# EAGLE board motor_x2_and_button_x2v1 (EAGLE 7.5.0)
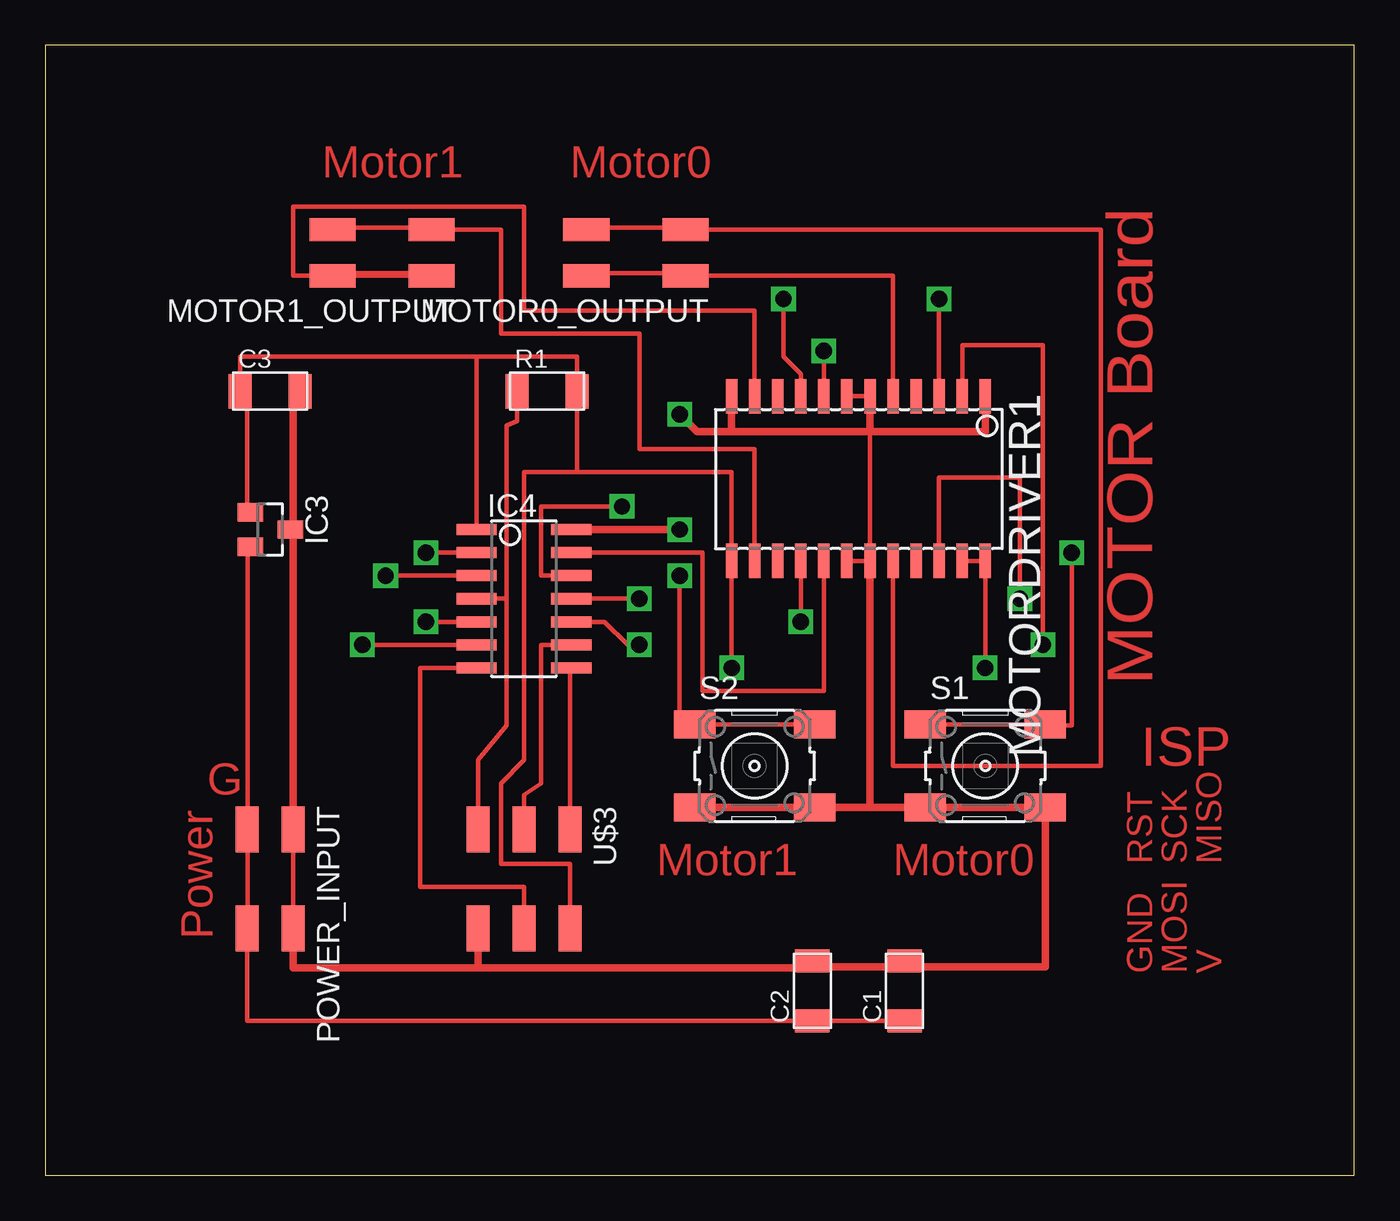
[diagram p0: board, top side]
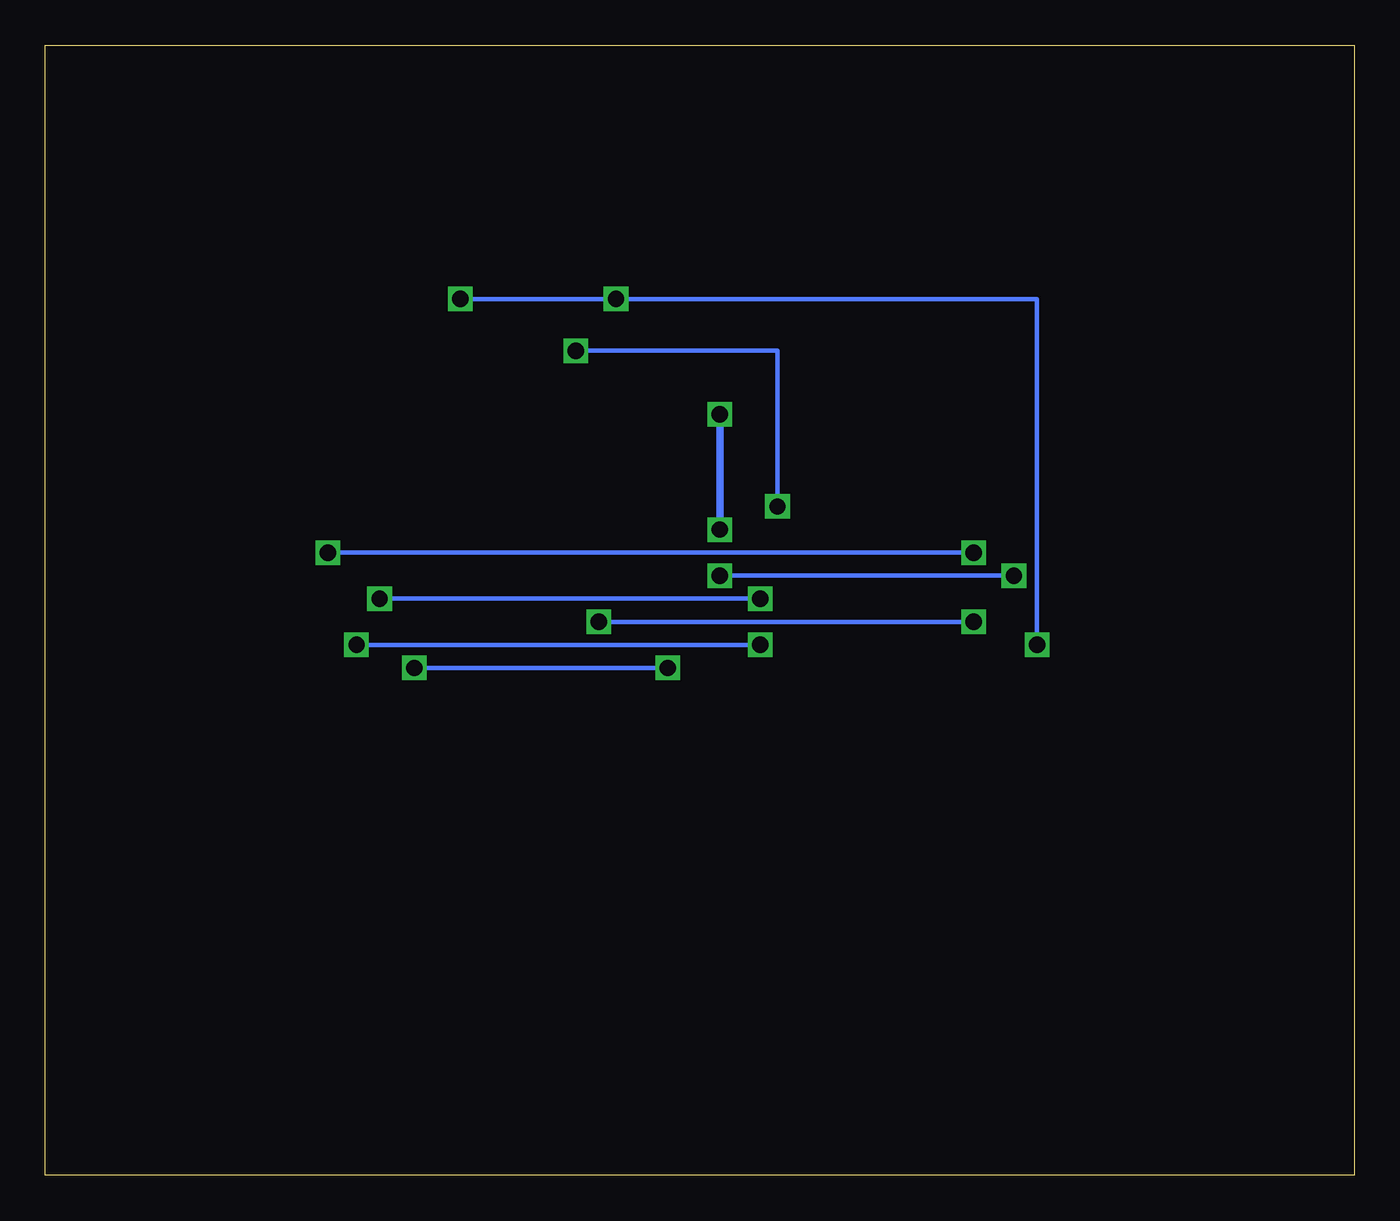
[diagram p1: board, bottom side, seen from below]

Size 72.06 x 62.22 mm. Coordinates in mm from the lower left corner, seen from the top.
Outline: 0,0 72.06,0 72.06,62.22 0,62.22 0,0
Copper layers (1*16): Top 0.035mm / dielectric 1.5mm / Bottom 0.035mm
Design rules "default": minimum track width 10mil, minimum drill 24mil, track to track 8mil, track to pad 8mil, pad to pad 8mil, via to via 8mil, smd to smd 8mil, copper to edge 40mil, drill to drill 8mil, minimum pad ring 10mil, minimum via ring 8mil, stop-mask expansion 4mil, vias tented up to drill 0mil, thermal gap 10mil

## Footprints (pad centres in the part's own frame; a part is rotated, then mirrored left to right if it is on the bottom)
C1206FAB = smd 1.27 x 1.905: 1 -1.651,0; 2 1.651,0
SOT23 = smd 1 x 1.4: 1 -0.95,-1.1; 2 0.95,-1.1; 3 0,1.1
SOIC14 = smd 0.61 x 2.21: 1 -3.81,-2.603; 2 -2.54,-2.603; 3 -1.27,-2.603; 4 0,-2.603; 5 1.27,-2.603; 6 2.54,-2.603; 7 3.81,-2.603; 8 3.81,2.603; 9 2.54,2.603; 10 1.27,2.603; 11 0,2.603; 12 -1.27,2.603; 13 -2.54,2.603; 14 -3.81,2.603
2X02SMD = smd 2.54 x 1.27: 1 -2.54,1.27; 2 2.92,1.27; 3 -2.54,-1.27; 4 2.92,-1.27
NJM2670 = smd 0.635 x 1.905: 1 -6.985,-3.531; 2 -5.715,-3.531; 3 -4.445,-3.531; 4 -3.175,-3.531; 5 -1.905,-3.531; 6 -0.635,-3.531; 7 0.635,-3.531; 8 1.905,-3.531; 9 3.175,-3.531; 10 4.445,-3.531; 11 5.715,-3.531; 12 6.985,-3.531; 13 6.985,5.531; 14 5.715,5.531; 15 4.445,5.531; 16 3.175,5.531; 17 1.905,5.531; 18 0.635,5.531; 19 -0.635,5.531; 20 -1.905,5.531; 21 -3.175,5.531; 22 -4.445,5.531; 23 -5.715,5.531; 24 -6.985,5.531
R1206FAB = smd 1.27 x 1.905: 1 -1.651,0; 2 1.651,0
6MM_SWITCH = smd 2.286 x 1.524: 1 -3.302,2.286; 2 3.302,2.286; 3 -3.302,-2.286; 4 3.302,-2.286
2X03SMD = smd 2.54 x 1.27: 1 -2.54,2.54; 2 2.92,2.54; 3 -2.54,0; 4 2.92,0; 5 -2.54,-2.54; 6 2.92,-2.54

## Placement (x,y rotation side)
C1  1uF  [C1206FAB]  47.31,10.16 90 top
C2  10uF  [C1206FAB]  42.23,10.16 90 top
C3  1uF  [C1206FAB]  12.38,43.18 0 top
IC3  5V  [SOT23]  12.38,35.56 270 top
IC4  ATTINY44-SSU  [SOIC14]  26.35,31.75 270 top
MOTOR0_OUTPUT  [2X02SMD]  32.7,50.8 180 top
MOTOR1_OUTPUT  [2X02SMD]  18.73,50.8 180 top
MOTORDRIVER1  NJM2670  [NJM2670]  44.77,39.37 180 top
POWER_INPUT  [2X02SMD]  12.38,16.51 270 top
R1  10k  [R1206FAB]  27.62,43.18 0 top
S1  0  [6MM_SWITCH]  51.75,22.54 0 top
S2  1  [6MM_SWITCH]  39.05,22.54 0 top
U$3  AVRISPSMD  [2X03SMD]  26.35,16.51 270 top

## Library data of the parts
C1-C3 IC3 MOTOR0_OUTPUT MOTOR1_OUTPUT POWER_INPUT R1 S1 S2 U$3 = fab
IC4 = HelloKamakura
MOTORDRIVER1 = mylib

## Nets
BUTTON0: IC4.2 S1.1 S1.2
BUTTON1: IC4.3 S2.1 S2.2
ENABLE: IC4.6 MOTORDRIVER1.3 MOTORDRIVER1.9
GND: C1.2 C2.2 C3.2 IC3.3 IC4.14 MOTORDRIVER1.1 MOTORDRIVER1.6 MOTORDRIVER1.7 MOTORDRIVER1.12 MOTORDRIVER1.18 MOTORDRIVER1.19 POWER_INPUT.1 POWER_INPUT.2 S1.3 S1.4 S2.3 S2.4 U$3.6
MISO: IC4.8 U$3.1
MOSI: IC4.7 U$3.4
MOTOR0-0: MOTOR0_OUTPUT.1 MOTOR0_OUTPUT.2 MOTORDRIVER1.5
MOTOR0-1: MOTOR0_OUTPUT.3 MOTOR0_OUTPUT.4 MOTORDRIVER1.20
MOTOR1-0: MOTOR1_OUTPUT.1 MOTOR1_OUTPUT.2 MOTORDRIVER1.11
MOTOR1-1: MOTOR1_OUTPUT.3 MOTOR1_OUTPUT.4 MOTORDRIVER1.14
PA0: IC4.13 MOTORDRIVER1.17
PA1: IC4.12 MOTORDRIVER1.8
PA2: IC4.11 MOTORDRIVER1.22
PA3: IC4.10 MOTORDRIVER1.2
RST: IC4.4 R1.1 U$3.5
SCK: IC4.9 U$3.3
TSDARM: IC4.5 MOTORDRIVER1.16
VBAT: C1.1 C2.1 IC3.2 POWER_INPUT.3 POWER_INPUT.4
VCC: C3.1 IC3.1 IC4.1 MOTORDRIVER1.13 MOTORDRIVER1.23 MOTORDRIVER1.24 R1.2 U$3.2

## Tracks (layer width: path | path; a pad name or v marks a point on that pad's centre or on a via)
BUTTON0  (via drill 0.9)
  Top 0.254: 23.81,34.29 IC4.2 v20.95,34.29 | 48.58,25.4 48.45,25.4 S1.1 S1.2 55.05,24.77 56.52,24.77 v56.52,34.29
  Bottom 0.254: v20.95,34.29 v56.52,34.29
BUTTON1  (via drill 0.9)
  Top 0.254: S2.2 S2.1 34.92,24.83 | 34.92,24.83 34.92,24.77 | 34.92,24.83 v34.92,33.02 | v18.73,33.02 IC4.3
  Bottom 0.254: v34.92,33.02 v18.73,33.02
ENABLE  (via drill 0.9)
  Top 0.254: v49.21,48.26 MOTORDRIVER1.3 | IC4.6 v17.46,29.21 | MOTORDRIVER1.9 41.59,44.13 40.64,45.09 v40.64,48.26
  Bottom 0.254: v49.21,48.26 v40.64,48.26 17.46,48.26 v17.46,29.21
GND  (via drill 0.9)
  Top 0.254: POWER_INPUT.1 POWER_INPUT.2 13.65,13.11 | 13.65,35.51 IC3.3 13.65,35.56 | C3.2 13.65,43.18 | MOTORDRIVER1.7 MOTORDRIVER1.6 | MOTORDRIVER1.18 MOTORDRIVER1.19 45.4,40.96
  Top 0.406: POWER_INPUT.1 13.65,35.51 | 13.65,35.56 13.65,43.18 | S2.3 S2.4 45.4,20.26 | 45.4,20.26 S1.3 S1.4 55.05,11.49 47.31,11.49 | MOTORDRIVER1.19 45.4,20.26 | MOTORDRIVER1.6 45.4,40.96 | 45.4,40.96 51.75,40.96 MOTORDRIVER1.1 | MOTORDRIVER1.12 37.78,40.96 | 37.78,40.96 45.4,40.96 | IC4.14 v34.92,35.56 | POWER_INPUT.2 13.65,11.43 23.81,11.43 | 23.81,11.43 42.23,11.43 42.23,11.49 | U$3.6 23.81,11.43 | 42.23,11.49 C2.2 | 42.23,11.49 47.31,11.49 | 47.31,11.49 C1.2 | 37.78,40.96 35.88,40.96 v34.92,41.91
  Bottom 0.406: v34.92,35.56 v34.92,41.91
MISO
  Top 0.254: 28.97,27.74 IC4.8 28.89,27.94 U$3.1 28.97,19.05
MOSI
  Top 0.254: U$3.4 26.35,15.88 20.64,15.88 20.64,27.94 IC4.7
MOTOR0-0
  Top 0.254: MOTOR0_OUTPUT.2 29.88,49.68 35.14,49.68 MOTOR0_OUTPUT.1 46.67,49.53 MOTORDRIVER1.5
MOTOR0-1
  Top 0.254: MOTOR0_OUTPUT.4 29.88,52.2 35.14,52.2 MOTOR0_OUTPUT.3 58.1,52.07 58.1,22.54 46.67,22.54 MOTORDRIVER1.20
MOTOR1-0
  Top 0.254: MOTOR1_OUTPUT.2 15.94,49.68 21.2,49.68 MOTOR1_OUTPUT.1 13.65,49.53 13.65,53.34 26.35,53.34 26.35,47.62 39.05,47.62 MOTORDRIVER1.11
MOTOR1-1
  Top 0.254: MOTOR1_OUTPUT.4 15.94,52.2 21.2,52.2 MOTOR1_OUTPUT.3 25.08,52.07 25.08,46.35 32.7,46.35 32.7,40.01 39.05,40.01 MOTORDRIVER1.14
PA0
  Top 0.254: IC4.13 36.2,34.29 36.2,26.67 42.86,26.67 MOTORDRIVER1.17
PA1  (via drill 0.9)
  Top 0.254: IC4.12 27.3,33.02 27.3,36.83 v31.75,36.83 | v42.86,45.4 MOTORDRIVER1.8
  Bottom 0.254: v31.75,36.83 31.75,45.4 v42.86,45.4
PA2  (via drill 0.9)
  Top 0.254: IC4.11 v32.7,31.75 | v53.66,31.75 53.66,38.42 49.21,38.42 MOTORDRIVER1.22
  Bottom 0.254: v32.7,31.75 v53.66,31.75
PA3  (via drill 0.9)
  Top 0.254: MOTORDRIVER1.2 50.48,45.72 54.93,45.72 v54.93,29.21 | v32.7,29.21 32.07,29.21 30.8,30.48 IC4.10
  Bottom 0.254: v54.93,29.21 v32.7,29.21
RST
  Top 0.254: U$3.5 23.81,22.86 25.4,24.77 25.4,31.75 | 25.4,31.75 IC4.4 | R1.1 25.97,41.53 25.4,41.27 25.4,31.75
SCK
  Top 0.254: U$3.3 26.35,20.95 27.3,21.59 27.3,29.21 IC4.9
TSDARM  (via drill 0.9)
  Top 0.254: IC4.5 v20.95,30.48 | v41.59,30.48 MOTORDRIVER1.16
  Bottom 0.254: v20.95,30.48 v41.59,30.48
VBAT
  Top 0.254: IC3.2 11.14,34.59 11.14,18.59 POWER_INPUT.3 11.14,18.36 11.14,13.11 POWER_INPUT.4 11.11,8.51 C2.1 C1.1
VCC  (via drill 0.9)
  Top 0.254: IC3.1 11.11,36.51 11.11,42.55 10.73,42.55 C3.1 10.73,45.09 23.75,45.09 | U$3.2 28.89,17.14 25.08,17.14 25.08,21.59 26.35,22.86 26.35,38.73 29.27,38.73 | 29.27,38.73 R1.2 29.27,45.09 23.75,45.09 | IC4.1 23.75,45.09 | 29.27,38.73 37.78,38.73 MOTORDRIVER1.13 v37.78,27.94 | MOTORDRIVER1.23 MOTORDRIVER1.24 v51.75,27.94
  Bottom 0.254: v37.78,27.94 v51.75,27.94

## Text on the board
Top: Motor1 | Motor0 | MOTOR Board | ISP | G | Motor1 | Motor0 | RST | SCK | MISO | Power | GND | MOSI | V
